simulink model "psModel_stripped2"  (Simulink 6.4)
settings: Solver=ode45  StartTime=psSimStruct.psSimPar.tStart  StopTime=psSimStruct.psSimPar.tStop  MaxStep=psSimStruct.psSimPar.maxStep  RelTol=psSimStruct.psSimPar.relTol
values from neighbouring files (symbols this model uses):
  psSimStruct = []    [psStartUp.m]
undefined symbols (not defined in the file or in its folder): psValve, psVolume, Restriction

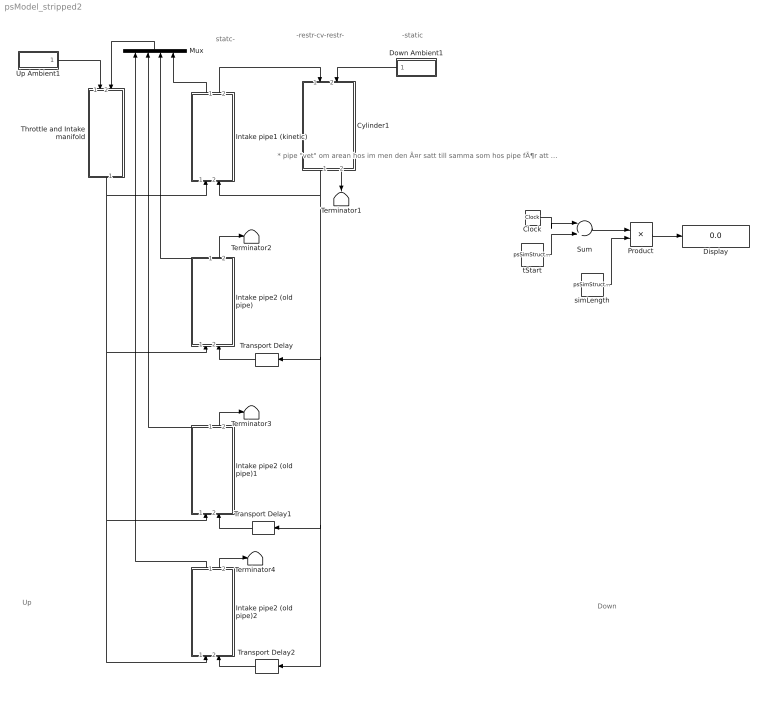
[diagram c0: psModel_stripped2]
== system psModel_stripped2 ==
  note: -restr-cv-restr-
  note: -static
  note: Down
  note: Up
  note: statc-
  note: * pipe "vet" om arean hos im men den Ã¤r satt till samma som hos pipe fÃ¶r att testa instabilitet * N_pipe har laggts till
  Clock : Clock
  Cylinder1 : Subsystem  Orientation=down  AncestorBlock=psModelLibrary/Cylinder  mask{thetaOffset=0, CylNbr=1}
      mask prompts: thetaOffset "thetaOffset [rad]"; CylNbr "Cylinder Number"
  Display : Display
  Down Ambient1 : Subsystem  Orientation=left
  Intake pipe1 (kinetic) : Subsystem  Orientation=up  AncestorBlock=psModelLibrary/Intake pipe
  Intake pipe2 (old pipe) : Subsystem  Orientation=up  AncestorBlock=psModelLibrary/Intake pipe
  Intake pipe2 (old pipe)1 : Subsystem  Orientation=up  AncestorBlock=psModelLibrary/Intake pipe
  Intake pipe2 (old pipe)2 : Subsystem  Orientation=up  AncestorBlock=psModelLibrary/Intake pipe
  Mux : Mux  Orientation=up
  Product : Product  Inputs=*/
  Sum : Sum  Inputs=|+-
  Terminator{1..4} (4 alike) : Terminator
  Throttle and Intake manifold : Subsystem  Orientation=down  mask{NumCyls=4}
      mask prompts: NumCyls "Number of Cylinders"
  Transport Delay : TransportDelay  Orientation=left  DelayTime=1/2/psSimStruct.psSimPar.RPS  InitialOutput=[0 psSimStruct.psModel.pIC_IM psSimStruct.psModel.TIC_IM psSimStruct.psModel.XgcIC_IM ]  BufferSize=10000
  Transport Delay1 : TransportDelay  Orientation=left  DelayTime=1/psSimStruct.psSimPar.RPS  InitialOutput=[0 psSimStruct.psModel.pIC_IM psSimStruct.psModel.TIC_IM psSimStruct.psModel.XgcIC_IM ]  BufferSize=10000
  Transport Delay2 : TransportDelay  Orientation=left  DelayTime=3/2/psSimStruct.psSimPar.RPS  InitialOutput=[0 psSimStruct.psModel.pIC_IM psSimStruct.psModel.TIC_IM psSimStruct.psModel.XgcIC_IM ]  BufferSize=10000
  Up Ambient1 : Subsystem
  simLength : Constant  Value=psSimStruct.psSimPar.tStop-psSimStruct.psSimPar.tStart
  tStart : Constant  Value=psSimStruct.psSimPar.tStart
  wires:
  Down Ambient1/1(out up) -> Cylinder1/2(in down)
  Cylinder1/2(out down) -> Terminator1/1
  Up Ambient1/1(out down) -> Throttle and Intake manifold/1(in up)
  Throttle and Intake manifold/1(out down) -> Intake pipe1 (kinetic)/1(in up), Intake pipe2 (old pipe)/1(in up), Intake pipe2 (old pipe)1/1(in up), Intake pipe2 (old pipe)2/1(in up)
  Cylinder1/1(out up) -> Intake pipe1 (kinetic)/2(in down), Transport Delay/1, Transport Delay1/1, Transport Delay2/1
  Intake pipe1 (kinetic)/2(out down) -> Cylinder1/1(in up)
  tStart/1 -> Sum/2
  Sum/1 -> Product/1
  simLength/1 -> Product/2
  Product/1 -> Display/1
  Clock/1 -> Sum/1
  Intake pipe2 (old pipe)/1(out up) -> Mux/3
  Intake pipe2 (old pipe)1/1(out up) -> Mux/2
  Intake pipe2 (old pipe)2/1(out up) -> Mux/1
  Transport Delay/1 -> Intake pipe2 (old pipe)/2(in down)
  Intake pipe2 (old pipe)/2(out down) -> Terminator2/1
  Transport Delay1/1 -> Intake pipe2 (old pipe)1/2(in down)
  Transport Delay2/1 -> Intake pipe2 (old pipe)2/2(in down)
  Intake pipe2 (old pipe)1/2(out down) -> Terminator3/1
  Intake pipe2 (old pipe)2/2(out down) -> Terminator4/1
  Mux/1 -> Throttle and Intake manifold/2(in down)
  Intake pipe1 (kinetic)/1(out up) -> Mux/4

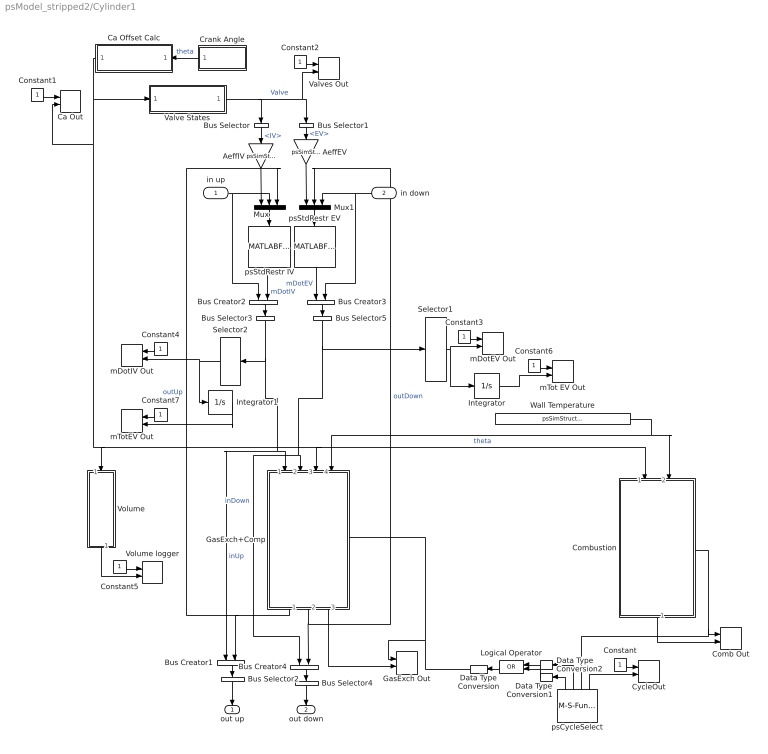
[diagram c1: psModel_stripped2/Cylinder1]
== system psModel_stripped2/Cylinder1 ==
  in up : Inport
  in down : Inport  Orientation=left  Port=2
  AeffEV : Gain  Orientation=down  Gain=psSimStruct.psGeometry.Ath_EV*psSimStruct.psGeometry.Cd_EV
  AeffIV : Gain  Orientation=down  Gain=psSimStruct.psGeometry.Ath_IV*psSimStruct.psGeometry.Cd_IV
  Bus Creator{1..4} (4 alike) : BusCreator  Orientation=down  Inputs=2
  Bus Selector : BusSelector  Orientation=down  OutputSignals=IV
  Bus Selector1 : BusSelector  Orientation=down  OutputSignals=EV
  Bus Selector2 : BusSelector  Orientation=down  OutputSignals=inUp.mDotIV,outUp.state  OutputAsBus=on
  Bus Selector3 : BusSelector  Orientation=down  OutputSignals=mDotIV,signal1.state  OutputAsBus=on
  Bus Selector4 : BusSelector  Orientation=down  OutputSignals=inDown.mDotEV,outDown.state  OutputAsBus=on
  Bus Selector5 : BusSelector  Orientation=down  OutputSignals=mDotEV,signal2.state  OutputAsBus=on
  Ca Offset Calc : Subsystem  Orientation=left
  Ca Out : M-S-Function  FunctionName=psToWorkspace  Parameters=1,int16('theta'),CylNbr
  Comb Out : M-S-Function  FunctionName=psToWorkspace  Parameters=9+2*psSimStruct.psThermProp.K,int16('pcb Vb Tb Vu Tu'),CylNbr
  Combustion : Subsystem  Orientation=down  TreatAsAtomicUnit=on
  Constant{,1..3,5..6} (6 alike) : Constant
  Constant4 : Constant  Orientation=left
  Constant7 : Constant  Orientation=left
  Crank Angle : Subsystem  Orientation=left
  CycleOut : M-S-Function  FunctionName=psToWorkspace  Parameters=1,int16('phase'),CylNbr
  Data Type Conversion : DataTypeConversion  Orientation=left
  Data Type Conversion1 : DataTypeConversion  Orientation=left
  Data Type Conversion2 : DataTypeConversion  Orientation=left
  GasExch Out : M-S-Function  FunctionName=psToWorkspace  Parameters=psSimStruct.psThermProp.K+4,int16('pge Vge Tge'),CylNbr
  GasExch+Comp : Subsystem  Orientation=down  Priority=1
  Integrator : Integrator
  Integrator1 : Integrator
  Logical Operator : Logic  Orientation=left  Operator=OR  AllPortsSameDT=off  OutDataTypeMode=Boolean  LogicDataType=uint
  Mux : Mux  Orientation=down  Inputs=3
  Mux1 : Mux  Orientation=down  Inputs=3
  Selector1 : Selector  Elements=[1]  Rows=[1]  OutputPortSize=[(-2)]
  Selector2 : Selector  Orientation=left  Elements=[1]  Rows=[1]  OutputPortSize=[(-2)]
  Valve States : Subsystem
  Valves Out : M-S-Function  FunctionName=psToWorkspace  Parameters=2,int16('uIV uEV'),CylNbr
  Volume : Subsystem  Orientation=down
  Volume logger : M-S-Function  FunctionName=psToWorkspace  Parameters=1,int16('V'),CylNbr
  Wall Temperature : Constant  Value=psSimStruct.psModel.T_Wall
  mDotEV Out : M-S-Function  FunctionName=psToWorkspace  Parameters=1,int16('mDotEV'),CylNbr
  mDotIV Out : M-S-Function  Orientation=left  FunctionName=psToWorkspace  Parameters=1,int16('mDotIV'),CylNbr
  mTot EV Out : M-S-Function  FunctionName=psToWorkspace  Parameters=1,int16('mTotEV'),CylNbr
  mTotEV Out : M-S-Function  Orientation=left  FunctionName=psToWorkspace  Parameters=1,int16('mTotIV'),CylNbr
  psCycleSelect : M-S-Function  Orientation=up  FunctionName=psCycleSelect  Parameters=caOffset  mask{caOffset=thetaOffset}
      mask prompts: caOffset "caOffset [rad]"
  psStdRestr EV : MATLABFcn  Orientation=down  MATLABFcn=psStdRestr  OutputDimensions=1  OutputSignalType=real
  psStdRestr IV : MATLABFcn  Orientation=down  MATLABFcn=psStdRestr  OutputDimensions=1  OutputSignalType=real
  out up : Outport  Orientation=down
  out down : Outport  Orientation=down  Port=2
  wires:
  Volume/1(V) -> Volume logger/2
  Constant5/1 -> Volume logger/1
  Selector2/1 -> mDotIV Out/2, Integrator1/1
  Selector1/1 -> mDotEV Out/2, Integrator/1
  in up/1 -> Mux/2, Bus Creator2/1
  Valve States/1("[iv ev]") -> Bus Selector/1, Bus Selector1/1, Valves Out/2  "Valve"
  AeffEV/1 -> Mux1/1
  AeffIV/1 -> Mux/1
  in down/1 -> Mux1/3, Bus Creator3/2
  psStdRestr EV/1 -> Bus Creator3/1  "mDotEV"
  Bus Selector1/1 -> AeffEV/1  "<EV>"
  Mux1/1 -> psStdRestr EV/1
  Bus Selector/1 -> AeffIV/1  "<IV>"
  Mux/1 -> psStdRestr IV/1
  Ca Offset Calc/1(theta out) -> Valve States/1(theta [rad]), Volume/1(theta in), GasExch+Comp/3(theta), Combustion/1(theta), Ca Out/2  "theta"
  Crank Angle/1(theta [rad]) -> Ca Offset Calc/1(theta in)  "theta"
  psStdRestr IV/1 -> Bus Creator2/2  "mDotIV"
  Bus Creator2/1 -> Bus Selector3/1
  Bus Creator3/1 -> Bus Selector5/1
  GasExch+Comp/2(out down) -> Mux1/2, Bus Creator4/2  "outDown"
  GasExch+Comp/1(out up) -> Mux/3, Bus Creator1/2  "outUp"
  Wall Temperature/1 -> Combustion/2(Wall Temperature), GasExch+Comp/4(T_Wall)
  Bus Selector3/1 -> Selector2/1, GasExch+Comp/1(inUp), Bus Creator1/1  "inUp"
  Bus Selector5/1 -> Selector1/1, GasExch+Comp/2(inDown), Bus Creator4/1  "inDown"
  psCycleSelect/3 -> Comb Out/1, Combustion/Enable
  Bus Creator1/1 -> Bus Selector2/1
  Bus Creator4/1 -> Bus Selector4/1
  GasExch+Comp/3(IntOut) -> GasExch Out/2
  Combustion/1(IntOut) -> Comb Out/2
  psCycleSelect/4 -> CycleOut/2
  Constant/1 -> CycleOut/1
  Constant1/1 -> Ca Out/1
  Constant2/1 -> Valves Out/1
  Constant3/1 -> mDotEV Out/1
  Constant4/1 -> mDotIV Out/1
  Bus Selector4/1 -> out down/1
  Bus Selector2/1 -> out up/1
  psCycleSelect/2 -> Data Type Conversion2/1
  psCycleSelect/1 -> Data Type Conversion1/1
  Logical Operator/1 -> Data Type Conversion/1
  Data Type Conversion/1 -> GasExch+Comp/Enable, GasExch Out/1
  Data Type Conversion1/1 -> Logical Operator/2
  Data Type Conversion2/1 -> Logical Operator/1
  Integrator/1 -> mTot EV Out/2
  Constant6/1 -> mTot EV Out/1
  Integrator1/1 -> mTotEV Out/2
  Constant7/1 -> mTotEV Out/1

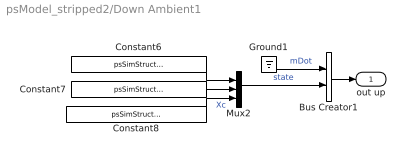
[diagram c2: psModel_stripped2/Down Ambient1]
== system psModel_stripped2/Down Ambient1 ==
  Bus Creator1 : BusCreator  Inputs=2
  Constant6 : Constant  Value=psSimStruct.psModel.pAmb
  Constant7 : Constant  Value=psSimStruct.psModel.TAmb
  Constant8 : Constant  Value=psSimStruct.psModel.XgcExh
  Ground1 : Ground
  Mux2 : Mux  Inputs=3
  out up : Outport
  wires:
  Ground1/1 -> Bus Creator1/1  "mDot"
  Mux2/1 -> Bus Creator1/2  "state"
  Constant7/1 -> Mux2/2
  Constant8/1 -> Mux2/3  "Xc"
  Bus Creator1/1 -> out up/1
  Constant6/1 -> Mux2/1

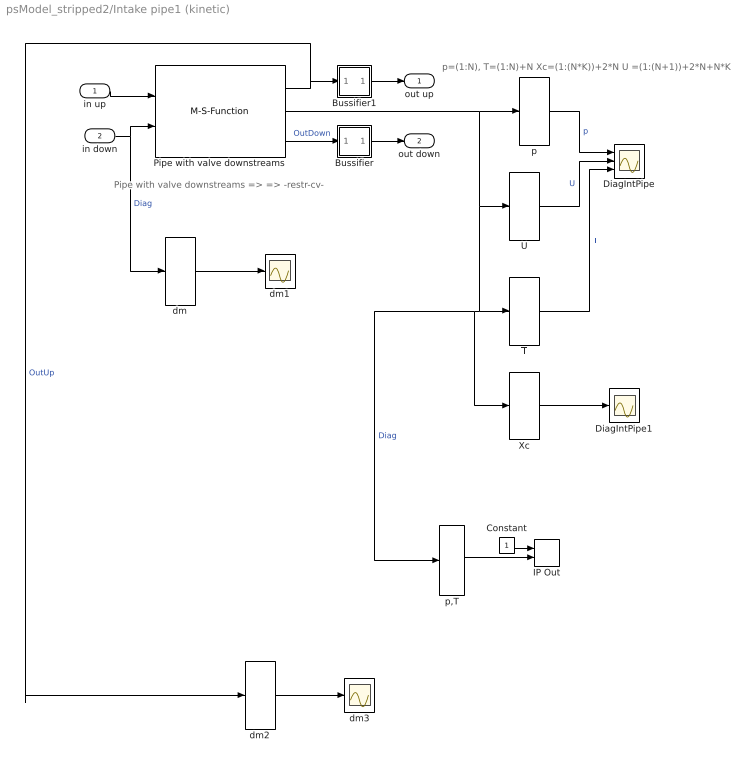
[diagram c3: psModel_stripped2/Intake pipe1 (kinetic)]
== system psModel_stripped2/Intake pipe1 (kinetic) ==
  note: Pipe with valve downstreams => => -restr-cv-
  note: p=(1:N), T=(1:N)+N Xc=(1:(N*K))+2*N U =(1:(N+1))+2*N+N*K
  in up : Inport
  in down : Inport  Port=2
  Bussifier : Subsystem
  Bussifier1 : Subsystem
  Constant : Constant
  DiagIntPipe : Scope  NumInputPorts=3
  DiagIntPipe1 : Scope
  IP Out : M-S-Function  FunctionName=psToWorkspace  Parameters=4,int16('pIP_U pIP_D TIP_U TIP_D'),1
  Pipe with valve downstreams : M-S-Function  FunctionName=psMultiGasPipe_Kinetic  Parameters=N,NumInputs,x,A,Pinit,Tinit,propInit,kFric,AUp,ADown,connectorUp,connectorDown  mask{N=psSimStruct.psModel.N_pipe, NumInputs=[1,1], x=psSimStruct.psModel.length_pipe_IM, A=psSimStruct.psModel.area_pipe_IM, Pinit=psSimStruct.psModel.pIC_IM, Tinit=psSimStruct.psModel.TIC_IM, propInit=psSimStruct.psModel.XgcIC_IM, kFric=psSimStruct.psModel.friction_IM, AUp=psSimStruct.psModel.area_pipe_IM, ADown=eps, connectorUp=Control Volume, connectorDown=Restriction}
      mask prompts: N "Number of elements"; NumInputs "Number of Inputs"; x "Pipe length [m]"; A "Pipe Area [m²]"; Pinit "Initial Pressure [Pa]"; Tinit "Initial Temperature [K]"; propInit "Initial prop [-]"; kFric "Pipe Friction"; AUp "Area of upstreams Pipe"; ADown "Area of downstreams Pipe"; connectorUp "Upstreams connector"; connectorDown "Downstreams connector"
  T : Selector  Elements=(1:psSimStruct.psModel.N_pipe)+psSimStruct.psModel.N_pipe  Rows=(1:3)+3  OutputPortSize=[(-2)]
  U : Selector  Elements=(1:(psSimStruct.psModel.N_pipe+1))+2*psSimStruct.psModel.N_pipe+psSimStruct.psModel.N_pipe*psSimStruct.psThermProp.K  Rows=(1:(3+1))+2*3+3*psSimStruct.psThermProp.K  OutputPortSize=[(-2)]
  Xc : Selector  Elements=2*psSimStruct.psModel.N_pipe+1:(psSimStruct.psModel.N_pipe*psSimStruct.psThermProp.K)  Rows=(1:3)+3  OutputPortSize=[(-2)]
  dm : Selector  Rows=(1:3)+3  OutputPortSize=[(-2)]
  dm1 : Scope
  dm2 : Selector  Rows=(1:3)+3  OutputPortSize=[(-2)]
  dm3 : Scope
  p : Selector  Elements=1:psSimStruct.psModel.N_pipe  Rows=1:3  OutputPortSize=[(-2)]
  p,T : Selector  Elements=[1 psSimStruct.psModel.N_pipe psSimStruct.psModel.N_pipe+1 2*psSimStruct.psModel.N_pipe]  Rows=[2 3]  OutputPortSize=[(-2)]
  out up : Outport
  out down : Outport  Port=2
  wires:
  U/1 -> DiagIntPipe/2  "U"
  Pipe with valve downstreams/2 -> p/1, U/1, T/1, p,T/1, Xc/1  "Diag"
  Pipe with valve downstreams/3 -> Bussifier/1(In1)  "OutDown"
  p/1 -> DiagIntPipe/1  "p"
  Bussifier1/1(Out1) -> out up/1
  Bussifier/1(Out1) -> out down/1
  Pipe with valve downstreams/1 -> Bussifier1/1(In1), dm2/1  "OutUp"
  in down/1 -> Pipe with valve downstreams/2, dm/1  "Diag"
  in up/1 -> Pipe with valve downstreams/1
  T/1 -> DiagIntPipe/3  "T"
  p,T/1 -> IP Out/2
  Constant/1 -> IP Out/1
  Xc/1 -> DiagIntPipe1/1
  dm/1 -> dm1/1
  dm2/1 -> dm3/1

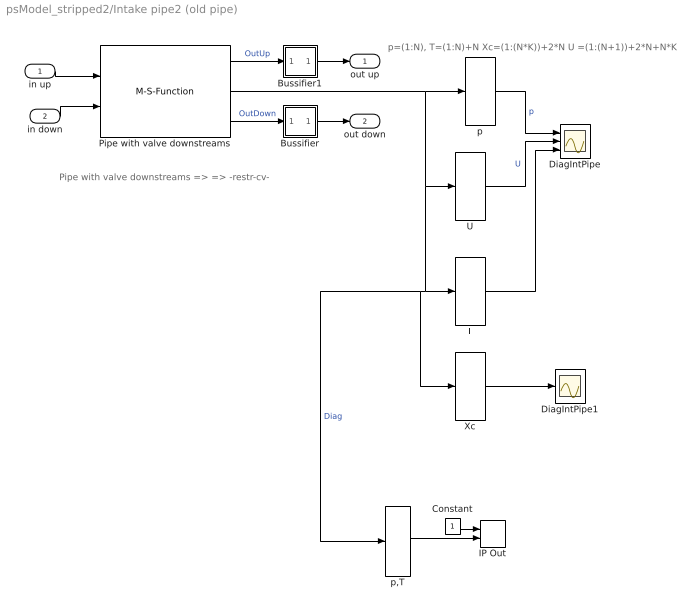
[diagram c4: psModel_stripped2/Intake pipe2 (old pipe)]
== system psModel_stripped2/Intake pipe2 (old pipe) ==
  note: p=(1:N), T=(1:N)+N Xc=(1:(N*K))+2*N U =(1:(N+1))+2*N+N*K
  note: Pipe with valve downstreams => => -restr-cv-
  in up : Inport
  in down : Inport  Port=2
  Bussifier : Subsystem
  Bussifier1 : Subsystem
  Constant : Constant
  DiagIntPipe : Scope  NumInputPorts=3
  DiagIntPipe1 : Scope
  IP Out : M-S-Function  FunctionName=psToWorkspace  Parameters=4,int16('pIP_U pIP_D TIP_U TIP_D'),2
  Pipe with valve downstreams : M-S-Function  FunctionName=psMultiGasPipe  Parameters=N,NumInputs,x,A,Pinit,Tinit,propInit,kFric,connectorUp,connectorDown  mask{N=3, NumInputs=[1,1], x=psSimStruct.psModel.length_pipe_IM, A=psSimStruct.psModel.area_pipe_IM, Pinit=psSimStruct.psModel.pIC_IM, Tinit=psSimStruct.psModel.TIC_IM, propInit=psSimStruct.psModel.XgcIC_IM, kFric=psSimStruct.psModel.friction_IM, connectorUp=Control Volume, connectorDown=Restriction}
      mask prompts: N "Number of elements"; NumInputs "Number of Inputs"; x "Pipe length [m]"; A "Pipe Area [m²]"; Pinit "Initial Pressure [Pa]"; Tinit "Initial Temperature [K]"; propInit "Initial prop [-]"; kFric "Pipe Friction"; connectorUp "Upstreams connector"; connectorDown "Downstreams connector"
  T : Selector  Elements=(1:3)+3  Rows=(1:3)+3  InputPortWidth=22  OutputPortSize=[(-2)]
  U : Selector  Elements=(1:(3+1))+2*3+3*psSimStruct.psThermProp.K  Rows=(1:(3+1))+2*3+3*psSimStruct.psThermProp.K  InputPortWidth=22  OutputPortSize=[(-2)]
  Xc : Selector  Elements="[15    16    17    18]"  Rows=(1:3)+3  InputPortWidth=22  OutputPortSize=[(-2)]
  p : Selector  Elements=1:3  Rows=1:3  InputPortWidth=22  OutputPortSize=[(-2)]
  p,T : Selector  Elements=[1 3 4 6]  Rows=[2 3]  OutputPortSize=[(-2)]
  out up : Outport
  out down : Outport  Port=2
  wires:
  Xc/1 -> DiagIntPipe1/1
  Constant/1 -> IP Out/1
  p,T/1 -> IP Out/2
  T/1 -> DiagIntPipe/3
  in up/1 -> Pipe with valve downstreams/1
  in down/1 -> Pipe with valve downstreams/2
  Pipe with valve downstreams/1 -> Bussifier1/1(In1)  "OutUp"
  Bussifier/1(Out1) -> out down/1
  Bussifier1/1(Out1) -> out up/1
  p/1 -> DiagIntPipe/1  "p"
  Pipe with valve downstreams/3 -> Bussifier/1(In1)  "OutDown"
  Pipe with valve downstreams/2 -> Xc/1, p,T/1, T/1, U/1, p/1  "Diag"
  U/1 -> DiagIntPipe/2  "U"

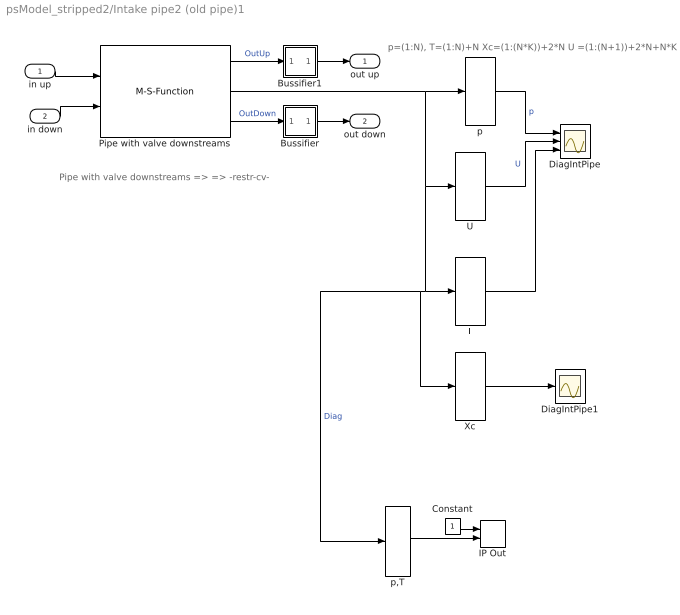
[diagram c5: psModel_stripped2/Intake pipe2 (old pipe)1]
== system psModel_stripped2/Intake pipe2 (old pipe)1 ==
  note: Pipe with valve downstreams => => -restr-cv-
  note: p=(1:N), T=(1:N)+N Xc=(1:(N*K))+2*N U =(1:(N+1))+2*N+N*K
  in up : Inport
  in down : Inport  Port=2
  Bussifier : Subsystem
  Bussifier1 : Subsystem
  Constant : Constant
  DiagIntPipe : Scope  NumInputPorts=3
  DiagIntPipe1 : Scope
  IP Out : M-S-Function  FunctionName=psToWorkspace  Parameters=4,int16('pIP_U pIP_D TIP_U TIP_D'),3
  Pipe with valve downstreams : M-S-Function  FunctionName=psMultiGasPipe  Parameters=N,NumInputs,x,A,Pinit,Tinit,propInit,kFric,connectorUp,connectorDown  mask{N=3, NumInputs=[1,1], x=psSimStruct.psModel.length_pipe_IM, A=psSimStruct.psModel.area_pipe_IM, Pinit=psSimStruct.psModel.pIC_IM, Tinit=psSimStruct.psModel.TIC_IM, propInit=psSimStruct.psModel.XgcIC_IM, kFric=psSimStruct.psModel.friction_IM, connectorUp=Control Volume, connectorDown=Restriction}
      mask prompts: N "Number of elements"; NumInputs "Number of Inputs"; x "Pipe length [m]"; A "Pipe Area [m²]"; Pinit "Initial Pressure [Pa]"; Tinit "Initial Temperature [K]"; propInit "Initial prop [-]"; kFric "Pipe Friction"; connectorUp "Upstreams connector"; connectorDown "Downstreams connector"
  T : Selector  Elements=(1:3)+3  Rows=(1:3)+3  InputPortWidth=22  OutputPortSize=[(-2)]
  U : Selector  Elements=(1:(3+1))+2*3+3*psSimStruct.psThermProp.K  Rows=(1:(3+1))+2*3+3*psSimStruct.psThermProp.K  InputPortWidth=22  OutputPortSize=[(-2)]
  Xc : Selector  Elements="[15    16    17    18]"  Rows=(1:3)+3  InputPortWidth=22  OutputPortSize=[(-2)]
  p : Selector  Elements=1:3  Rows=1:3  InputPortWidth=22  OutputPortSize=[(-2)]
  p,T : Selector  Elements=[1 3 4 6]  Rows=[2 3]  OutputPortSize=[(-2)]
  out up : Outport
  out down : Outport  Port=2
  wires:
  U/1 -> DiagIntPipe/2  "U"
  Pipe with valve downstreams/2 -> p/1, U/1, T/1, p,T/1, Xc/1  "Diag"
  Pipe with valve downstreams/3 -> Bussifier/1(In1)  "OutDown"
  p/1 -> DiagIntPipe/1  "p"
  Bussifier1/1(Out1) -> out up/1
  Bussifier/1(Out1) -> out down/1
  Pipe with valve downstreams/1 -> Bussifier1/1(In1)  "OutUp"
  in down/1 -> Pipe with valve downstreams/2
  in up/1 -> Pipe with valve downstreams/1
  T/1 -> DiagIntPipe/3
  p,T/1 -> IP Out/2
  Constant/1 -> IP Out/1
  Xc/1 -> DiagIntPipe1/1

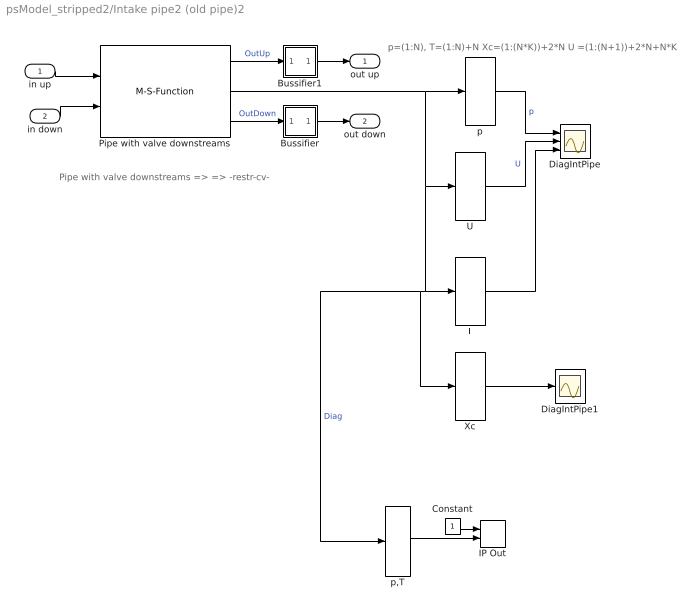
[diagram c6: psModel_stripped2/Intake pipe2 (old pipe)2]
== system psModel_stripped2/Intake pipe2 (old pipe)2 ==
  note: p=(1:N), T=(1:N)+N Xc=(1:(N*K))+2*N U =(1:(N+1))+2*N+N*K
  note: Pipe with valve downstreams => => -restr-cv-
  in up : Inport
  in down : Inport  Port=2
  Bussifier : Subsystem
  Bussifier1 : Subsystem
  Constant : Constant
  DiagIntPipe : Scope  NumInputPorts=3
  DiagIntPipe1 : Scope
  IP Out : M-S-Function  FunctionName=psToWorkspace  Parameters=4,int16('pIP_U pIP_D TIP_U TIP_D'),4
  Pipe with valve downstreams : M-S-Function  FunctionName=psMultiGasPipe  Parameters=N,NumInputs,x,A,Pinit,Tinit,propInit,kFric,connectorUp,connectorDown  mask{N=3, NumInputs=[1,1], x=psSimStruct.psModel.length_pipe_IM, A=psSimStruct.psModel.area_pipe_IM, Pinit=psSimStruct.psModel.pIC_IM, Tinit=psSimStruct.psModel.TIC_IM, propInit=psSimStruct.psModel.XgcIC_IM, kFric=psSimStruct.psModel.friction_IM, connectorUp=Control Volume, connectorDown=Restriction}
      mask prompts: N "Number of elements"; NumInputs "Number of Inputs"; x "Pipe length [m]"; A "Pipe Area [m²]"; Pinit "Initial Pressure [Pa]"; Tinit "Initial Temperature [K]"; propInit "Initial prop [-]"; kFric "Pipe Friction"; connectorUp "Upstreams connector"; connectorDown "Downstreams connector"
  T : Selector  Elements=(1:3)+3  Rows=(1:3)+3  InputPortWidth=22  OutputPortSize=[(-2)]
  U : Selector  Elements=(1:(3+1))+2*3+3*psSimStruct.psThermProp.K  Rows=(1:(3+1))+2*3+3*psSimStruct.psThermProp.K  InputPortWidth=22  OutputPortSize=[(-2)]
  Xc : Selector  Elements="[15    16    17    18]"  Rows=(1:3)+3  InputPortWidth=22  OutputPortSize=[(-2)]
  p : Selector  Elements=1:3  Rows=1:3  InputPortWidth=22  OutputPortSize=[(-2)]
  p,T : Selector  Elements=[1 3 4 6]  Rows=[2 3]  OutputPortSize=[(-2)]
  out up : Outport
  out down : Outport  Port=2
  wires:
  Xc/1 -> DiagIntPipe1/1
  Constant/1 -> IP Out/1
  p,T/1 -> IP Out/2
  T/1 -> DiagIntPipe/3
  in up/1 -> Pipe with valve downstreams/1
  in down/1 -> Pipe with valve downstreams/2
  Pipe with valve downstreams/1 -> Bussifier1/1(In1)  "OutUp"
  Bussifier/1(Out1) -> out down/1
  Bussifier1/1(Out1) -> out up/1
  p/1 -> DiagIntPipe/1  "p"
  Pipe with valve downstreams/3 -> Bussifier/1(In1)  "OutDown"
  Pipe with valve downstreams/2 -> Xc/1, p,T/1, T/1, U/1, p/1  "Diag"
  U/1 -> DiagIntPipe/2  "U"

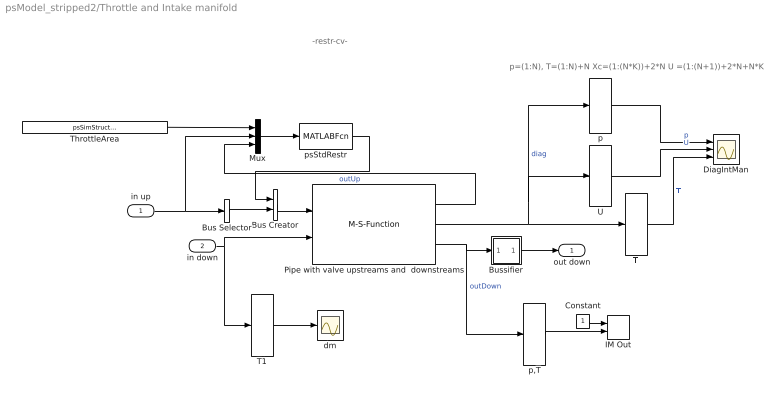
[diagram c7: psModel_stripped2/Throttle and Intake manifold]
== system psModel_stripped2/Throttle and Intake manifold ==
  note: -restr-cv-
  note: p=(1:N), T=(1:N)+N Xc=(1:(N*K))+2*N U =(1:(N+1))+2*N+N*K
  in up : Inport
  in down : Inport  Port=2
  Bus Creator : BusCreator  Inputs=2
  Bus Selector : BusSelector  OutputSignals=state  OutputAsBus=on
  Bussifier : Subsystem
  Constant : Constant
  DiagIntMan : Scope  NumInputPorts=3
  IM Out : M-S-Function  FunctionName=psToWorkspace  Parameters=2,int16('pIM TIM'),1
  Mux : Mux  Inputs=3
  Pipe with valve upstreams and  downstreams : M-S-Function  FunctionName=psMultiGasPipe  Parameters=N,NumInputs,x,A,Pinit,Tinit,propInit,kFric,connectorUp,connectorDown  mask{N=1, NumInputs=[1,NumCyls], x=psSimStruct.psModel.length_common_IM, A=psSimStruct.psModel.area_common_IM, Pinit=psSimStruct.psModel.pIC_IM, Tinit=psSimStruct.psModel.TIC_IM, propInit=psSimStruct.psModel.XgcIC_IM, kFric=psSimStruct.psModel.friction_IM, connectorUp=Restriction, connectorDown=Restriction}
      mask prompts: N "Number of elements"; NumInputs "Number of Inputs"; x "Pipe length [m]"; A "Pipe Area [m²]"; Pinit "Initial Pressure [Pa]"; Tinit "Initial Temperature [K]"; propInit "Initial prop [-]"; kFric "Pipe Friction"; connectorUp "Upstreams connector"; connectorDown "Downstreams connector"
  T : Selector  Elements=(1:1)+1  Rows=1:2+1  OutputPortSize=[(-2)]
  T1 : Selector  Rows=1:2+1  OutputPortSize=[(-2)]
  ThrottleArea : Constant  Value=psSimStruct.psModel.ThrottleArea
  U : Selector  Elements=(1:2)+2+psSimStruct.psThermProp.K  Rows=(1:2)+2+psSimStruct.psThermProp.K  OutputPortSize=[(-2)]
  dm : Scope
  p : Selector  Rows=[1 ]  OutputPortSize=[(-2)]
  p,T : Selector  Elements=[2 3]  Rows=[2 3]  OutputPortSize=[(-2)]
  psStdRestr : MATLABFcn  MATLABFcn=psStdRestr  OutputDimensions=1  OutputSignalType=real
  out down : Outport
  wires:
  p,T/1 -> IM Out/2
  Constant/1 -> IM Out/1
  Bussifier/1(Out1) -> out down/1
  Bus Selector/1 -> Bus Creator/2
  psStdRestr/1 -> Bus Creator/1
  Bus Creator/1 -> Pipe with valve upstreams and  downstreams/1
  Pipe with valve upstreams and  downstreams/1 -> Mux/3  "outUp"
  ThrottleArea/1 -> Mux/1
  in down/1 -> Pipe with valve upstreams and  downstreams/2, T1/1
  Mux/1 -> psStdRestr/1
  in up/1 -> Bus Selector/1, Mux/2
  Pipe with valve upstreams and  downstreams/3 -> Bussifier/1(In1), p,T/1  "outDown"
  Pipe with valve upstreams and  downstreams/2 -> p/1, U/1, T/1  "diag"
  U/1 -> DiagIntMan/2  "U"
  p/1 -> DiagIntMan/1  "p"
  T/1 -> DiagIntMan/3  "T"
  T1/1 -> dm/1

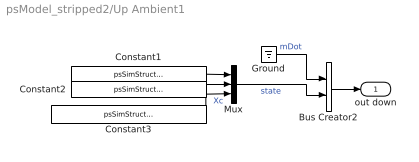
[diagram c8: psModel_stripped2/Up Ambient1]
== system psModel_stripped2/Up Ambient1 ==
  Bus Creator2 : BusCreator  Inputs=2
  Constant1 : Constant  Value=psSimStruct.psModel.pAmb
  Constant2 : Constant  Value=psSimStruct.psModel.TAmb
  Constant3 : Constant  Value=psSimStruct.psModel.XgcAmb
  Ground : Ground
  Mux : Mux  Inputs=3
  out down : Outport
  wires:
  Bus Creator2/1 -> out down/1
  Ground/1 -> Bus Creator2/1  "mDot"
  Mux/1 -> Bus Creator2/2  "state"
  Constant1/1 -> Mux/1
  Constant2/1 -> Mux/2
  Constant3/1 -> Mux/3  "Xc"

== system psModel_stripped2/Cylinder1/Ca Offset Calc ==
  theta in : Inport
  Sum : Sum  Inputs=|++
  thetaOffset : Constant  Value=thetaOffset
  theta out : Outport
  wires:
  Sum/1 -> theta out/1
  theta in/1 -> Sum/1
  thetaOffset/1 -> Sum/2

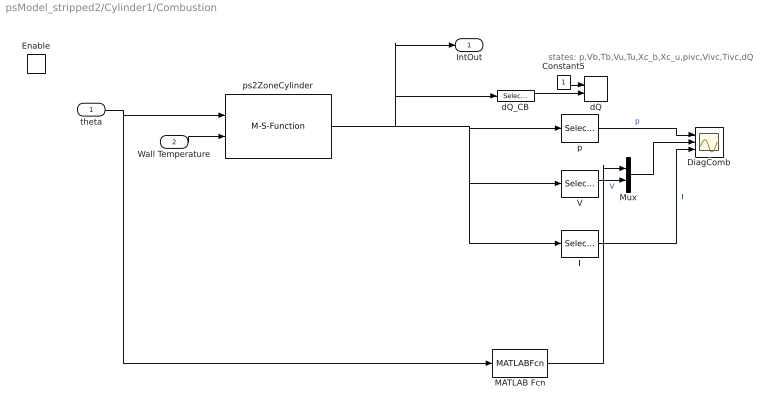
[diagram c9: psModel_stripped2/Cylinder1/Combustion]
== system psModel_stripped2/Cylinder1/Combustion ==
  note: states: p,Vb,Tb,Vu,Tu,Xc_b,Xc_u,pivc,Vivc,Tivc,dQ
  theta : Inport
  Wall Temperature : Inport  Port=2
  Enable : EnablePort  Orientation=left  StatesWhenEnabling=reset
  Constant5 : Constant
  DiagComb : Scope  NumInputPorts=3
  MATLAB Fcn : MATLABFcn  MATLABFcn=psVolume(u(1))  OutputDimensions=1
  Mux : Mux  Inputs=2
  T : Selector  Elements=[3 5]  Rows=[3 5]  OutputPortSize=[(-2)]
  V : Selector  Elements=[2 4]  Rows=[2 4]  OutputPortSize=[(-2)]
  dQ : M-S-Function  FunctionName=psToWorkspace  Parameters=1,int16('dQ'),CylNbr
  dQ_CB : Selector  Elements=[psSimStruct.psThermProp.K*2+9]  Rows=[psSimStruct.psThermProp.K*2+9]  OutputPortSize=[(-2)]
  p : Selector  Elements=[1]  Rows=[1]  OutputPortSize=[(-2)]
  ps2ZoneCylinder : M-S-Function  FunctionName=ps2ZoneCylinder  Parameters=thetaOffset,CylNbr
  IntOut : Outport
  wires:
  dQ_CB/1 -> dQ/2
  Constant5/1 -> dQ/1
  ps2ZoneCylinder/1 -> dQ_CB/1, IntOut/1, p/1, V/1, T/1
  p/1 -> DiagComb/1  "p"
  T/1 -> DiagComb/3  "T"
  V/1 -> Mux/2  "V"
  Mux/1 -> DiagComb/2
  MATLAB Fcn/1 -> Mux/1
  theta/1 -> MATLAB Fcn/1, ps2ZoneCylinder/1
  Wall Temperature/1 -> ps2ZoneCylinder/2

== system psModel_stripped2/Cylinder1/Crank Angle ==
  simulation time : Clock
  speed : Gain  Gain=psSimStruct.psSimPar.w
  theta [rad] : Outport
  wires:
  speed/1 -> theta [rad]/1
  simulation time/1 -> speed/1

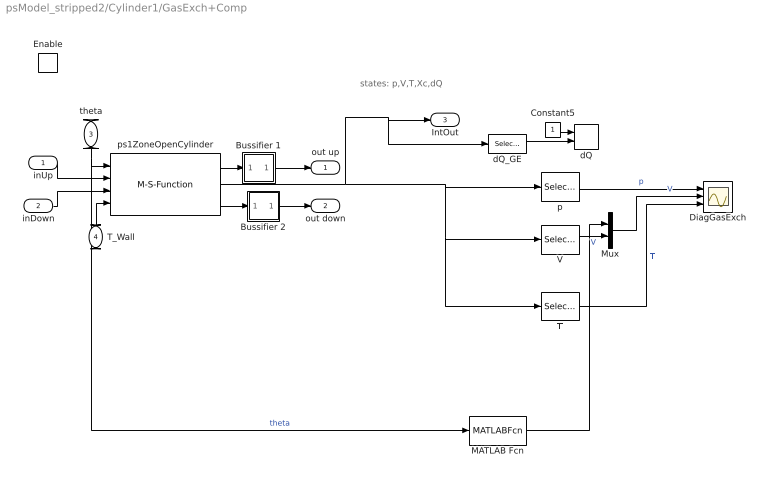
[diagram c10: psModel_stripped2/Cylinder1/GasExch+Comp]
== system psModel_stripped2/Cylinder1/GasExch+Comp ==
  note: states: p,V,T,Xc,dQ
  inUp : Inport
  inDown : Inport  Port=2
  theta : Inport  Orientation=down  Port=3
  T_Wall : Inport  Orientation=up  Port=4
  Enable : EnablePort  Orientation=left  StatesWhenEnabling=reset
  Bussifier 1 : Subsystem
  Bussifier 2 : Subsystem
  Constant5 : Constant
  DiagGasExch : Scope  NumInputPorts=3
  MATLAB Fcn : MATLABFcn  MATLABFcn=psVolume(u(1))  OutputDimensions=1
  Mux : Mux  Inputs=2
  T : Selector  Elements=[3]  Rows=[3]  OutputPortSize=[(-2)]
  V : Selector  Elements=[2]  Rows=[2]  OutputPortSize=[(-2)]
  dQ : M-S-Function  FunctionName=psToWorkspace  Parameters=1,int16('dQ'),CylNbr
  dQ_GE : Selector  Elements=[psSimStruct.psThermProp.K+4]  Rows=[psSimStruct.psThermProp.K+4]  OutputPortSize=[(-2)]
  p : Selector  Elements=[1]  Rows=[1]  OutputPortSize=[(-2)]
  ps1ZoneOpenCylinder : M-S-Function  FunctionName=ps1ZoneOpenCylinder  Parameters=thetaOffset,CylNbr
  out up : Outport  InitialOutput=[0 1e5 300 psSimStruct.psModel.XgcAmb]
  out down : Outport  Port=2  InitialOutput=[0 1e5 300 psSimStruct.psModel.XgcAmb]
  IntOut : Outport  Port=3
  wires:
  dQ_GE/1 -> dQ/2
  Constant5/1 -> dQ/1
  Bussifier 1/1(Out1) -> out up/1
  Bussifier 2/1(Out1) -> out down/1
  T_Wall/1 -> ps1ZoneOpenCylinder/4
  theta/1 -> ps1ZoneOpenCylinder/1, MATLAB Fcn/1  "theta"
  inUp/1 -> ps1ZoneOpenCylinder/2
  inDown/1 -> ps1ZoneOpenCylinder/3
  ps1ZoneOpenCylinder/1 -> Bussifier 1/1(In1)
  ps1ZoneOpenCylinder/3 -> Bussifier 2/1(In1)
  ps1ZoneOpenCylinder/2 -> dQ_GE/1, IntOut/1, p/1, T/1, V/1
  p/1 -> DiagGasExch/1  "p"
  T/1 -> DiagGasExch/3  "T"
  V/1 -> Mux/2  "V"
  Mux/1 -> DiagGasExch/2  "V"
  MATLAB Fcn/1 -> Mux/1

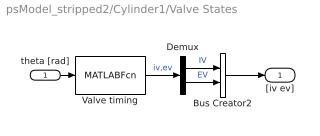
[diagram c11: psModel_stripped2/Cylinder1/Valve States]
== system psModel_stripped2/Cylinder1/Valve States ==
  theta [rad] : Inport
  Bus Creator2 : BusCreator  Inputs=2
  Demux : Demux  Outputs=2
  Valve timing : MATLABFcn  Description=|  MATLABFcn=psValve(u(1))  OutputDimensions=2
      | [u] = psValve(CA)                                   
      | Calculates the valve states. u = [u1 u2]', where u1  
      | is the intake valve and u2 the outlet valve.         
      | u1, u2 = 1 means fully open, u1, u2 = 0 means closed.
  "[iv ev]" : Outport
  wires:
  Valve timing/1 -> Demux/1  "iv,ev"
  Bus Creator2/1 -> "[iv ev]"/1
  Demux/2 -> Bus Creator2/2  "EV"
  Demux/1 -> Bus Creator2/1  "IV"
  theta [rad]/1 -> Valve timing/1

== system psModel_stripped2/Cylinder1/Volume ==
  theta in : Inport
  Total Volume : MATLABFcn  Description=|  MATLABFcn=psVolume(u(1))  OutputDimensions=1
      | [u] = psValve(CA)                                   
      | Calculates the valve states. u = [u1 u2]', where u1  
      | is the intake valve and u2 the outlet valve.         
      | u1, u2 = 1 means fully open, u1, u2 = 0 means closed.
  V : Outport
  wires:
  Total Volume/1 -> V/1
  theta in/1 -> Total Volume/1

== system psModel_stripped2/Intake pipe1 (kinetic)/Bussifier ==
  In1 : Inport
  Bus Creator1 : BusCreator  Inputs=2
  Demux : Demux  Outputs=[1 2+psSimStruct.psThermProp.K]
  Out1 : Outport
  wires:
  In1/1 -> Demux/1
  Bus Creator1/1 -> Out1/1
  Demux/2 -> Bus Creator1/2  "state"
  Demux/1 -> Bus Creator1/1  "mDot"

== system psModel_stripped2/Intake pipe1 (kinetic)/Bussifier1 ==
  In1 : Inport
  Bus Creator1 : BusCreator  Inputs=2
  Demux : Demux  Outputs=[1 2+psSimStruct.psThermProp.K]
  Out1 : Outport
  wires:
  Demux/1 -> Bus Creator1/1  "mDot"
  Demux/2 -> Bus Creator1/2  "state"
  Bus Creator1/1 -> Out1/1
  In1/1 -> Demux/1

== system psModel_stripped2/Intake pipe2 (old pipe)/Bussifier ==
  In1 : Inport
  Bus Creator1 : BusCreator  Inputs=2
  Demux : Demux  Outputs=[1 2+psSimStruct.psThermProp.K]
  Out1 : Outport
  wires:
  Demux/1 -> Bus Creator1/1  "mDot"
  Demux/2 -> Bus Creator1/2  "state"
  Bus Creator1/1 -> Out1/1
  In1/1 -> Demux/1

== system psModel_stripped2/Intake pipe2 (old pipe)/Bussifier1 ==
  In1 : Inport
  Bus Creator1 : BusCreator  Inputs=2
  Demux : Demux  Outputs=[1 2+psSimStruct.psThermProp.K]
  Out1 : Outport
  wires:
  In1/1 -> Demux/1
  Bus Creator1/1 -> Out1/1
  Demux/2 -> Bus Creator1/2  "state"
  Demux/1 -> Bus Creator1/1  "mDot"

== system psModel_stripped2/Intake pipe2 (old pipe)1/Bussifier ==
  In1 : Inport
  Bus Creator1 : BusCreator  Inputs=2
  Demux : Demux  Outputs=[1 2+psSimStruct.psThermProp.K]
  Out1 : Outport
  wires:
  In1/1 -> Demux/1
  Bus Creator1/1 -> Out1/1
  Demux/2 -> Bus Creator1/2  "state"
  Demux/1 -> Bus Creator1/1  "mDot"

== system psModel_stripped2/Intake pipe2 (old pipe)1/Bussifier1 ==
  In1 : Inport
  Bus Creator1 : BusCreator  Inputs=2
  Demux : Demux  Outputs=[1 2+psSimStruct.psThermProp.K]
  Out1 : Outport
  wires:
  Demux/1 -> Bus Creator1/1  "mDot"
  Demux/2 -> Bus Creator1/2  "state"
  Bus Creator1/1 -> Out1/1
  In1/1 -> Demux/1

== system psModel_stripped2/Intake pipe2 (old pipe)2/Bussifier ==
  In1 : Inport
  Bus Creator1 : BusCreator  Inputs=2
  Demux : Demux  Outputs=[1 2+psSimStruct.psThermProp.K]
  Out1 : Outport
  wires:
  Demux/1 -> Bus Creator1/1  "mDot"
  Demux/2 -> Bus Creator1/2  "state"
  Bus Creator1/1 -> Out1/1
  In1/1 -> Demux/1

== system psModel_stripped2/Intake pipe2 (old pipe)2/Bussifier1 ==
  In1 : Inport
  Bus Creator1 : BusCreator  Inputs=2
  Demux : Demux  Outputs=[1 2+psSimStruct.psThermProp.K]
  Out1 : Outport
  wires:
  In1/1 -> Demux/1
  Bus Creator1/1 -> Out1/1
  Demux/2 -> Bus Creator1/2  "state"
  Demux/1 -> Bus Creator1/1  "mDot"

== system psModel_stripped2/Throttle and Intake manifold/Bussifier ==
  In1 : Inport
  Bus Creator1 : BusCreator  Inputs=2
  Demux : Demux  Outputs=[1 2+psSimStruct.psThermProp.K]
  Out1 : Outport
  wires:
  In1/1 -> Demux/1
  Bus Creator1/1 -> Out1/1
  Demux/2 -> Bus Creator1/2  "state"
  Demux/1 -> Bus Creator1/1  "mDot"

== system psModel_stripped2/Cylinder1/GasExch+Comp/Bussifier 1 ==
  In1 : Inport
  Bus Creator2 : BusCreator  Inputs=2
  Ground : Ground
  Out1 : Outport
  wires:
  Bus Creator2/1 -> Out1/1
  In1/1 -> Bus Creator2/2  "state"
  Ground/1 -> Bus Creator2/1  "mDot"

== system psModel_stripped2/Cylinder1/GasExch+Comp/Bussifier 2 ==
  In1 : Inport
  Bus Creator2 : BusCreator  Inputs=2
  Ground : Ground
  Out1 : Outport
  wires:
  Ground/1 -> Bus Creator2/1  "mDot"
  In1/1 -> Bus Creator2/2  "state"
  Bus Creator2/1 -> Out1/1
